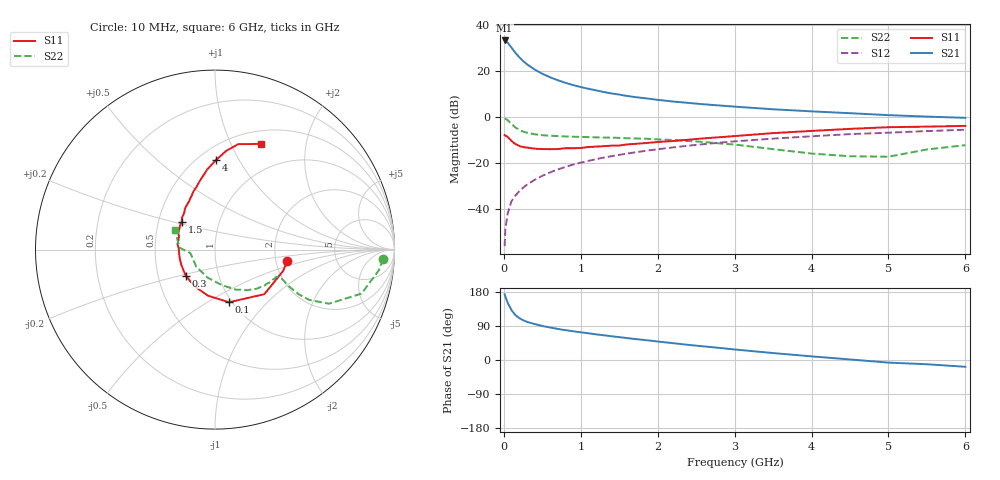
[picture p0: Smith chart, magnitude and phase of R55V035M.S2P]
! SIEMENS Small Signal Semiconductors
! BFR183
! Si NPN RF Bipolar Junction Transistor in SOT23
! VCE = 5 V  IC = 35 mA
! Common Emitter S-Parameters:  May  1996
# GHz  S  MA  R  50
!  f  S11  S21  S12  S22
! GHz  MAG  ANG  MAG  ANG  MAG  ANG  MAG  ANG
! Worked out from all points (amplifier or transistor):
!   36 points, 10 MHz to 6 GHz, reference 50 ohm
!   highest |S21| = 33.1 dB at 10 MHz (marker M1)
!   |S21| within 3 dB of that: start of sweep to 96.56 MHz
!   unconditionally stable (mu >= 1): 427.4 MHz to 2.37 GHz
!   at 250 MHz: K = 0.90, MSG = 27.4 dB, |S12| = -30.6 dB
!   at 1.4 GHz: K = 1.04, MAG = 12.3 dB, |S12| = -17.0 dB
!   at 6 GHz: K = 0.90, MSG = 2.6 dB, |S12| = -5.5 dB
!   S11 on the Smith chart (normalised r, x): 10 MHz: 2.31, -0.35; 100 MHz: 0.97, -0.63; 300 MHz: 0.69, -0.21; 1.5 GHz: 0.66, +0.22; 4 GHz: 0.61, +0.81; 6 GHz: 0.65, +1.31
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0.01  0.4074 -8.8  45.44 173.2  0.0016 85.1  0.9379 -3.2
0.02  0.398 -17.4  44.7 167.2  0.0038 76.1  0.9209 -7.1
0.05  0.3705 -42.1  40.73 151.0  0.0082 77.2  0.8527 -16.7
0.1  0.3036 -75.1  31.61 131.3  0.0151 73.8  0.7025 -25.4
0.15  0.2597 -98.6  24.54 118.6  0.0199 71.7  0.5954 -28.1
0.2  0.2365 -115.2  19.75 110.7  0.0248 71.9  0.5285 -28.1
0.25  0.2236 -128.2  16.33 105.0  0.0294 71.7  0.4847 -27.1
0.3  0.2184 -138.4  13.89 100.8  0.0343 73.4  0.4575 -26.3
0.4  0.2064 -154.6  10.69 94.9  0.0435 74.1  0.4231 -24.5
0.5  0.2026 -165.5  8.627 89.8  0.0534 75.0  0.4041 -23.5
0.6  0.2013 -174.2  7.26 85.8  0.0633 74.4  0.3939 -23.2
0.7  0.2027 177.1  6.273 82.1  0.0731 74.1  0.386 -23.4
0.8  0.2109 172.0  5.501 78.8  0.0831 73.3  0.3796 -23.6
0.9  0.2107 165.5  4.916 75.8  0.0932 72.8  0.3738 -24.1
1.1  0.2243 155.7  4.083 70.5  0.1124 71.1  0.3674 -26.5
1.5  0.2411 140.1  3.057 60.4  0.1516 67.1  0.3534 -31.5
2.2  0.3026 119.0  2.164 44.4  0.22 59.2  0.3178 -43.4
3.5  0.4483 95.6  1.471 18.3  0.3404 42.4  0.2017 -78.9
4  0.5001 89.2  1.326 9.6  0.3829 36.4  0.1618 -104.6
4.5  0.5538 83.5  1.21 1.4  0.4261 29.6  0.1415 -137.3
5.5  0.6192 71.7  1.021 -11.2  0.4964 18.0  0.1983 176.7
6  0.6428 66.5  0.96 -17.9  0.5299 10.4  0.2464 154.4
